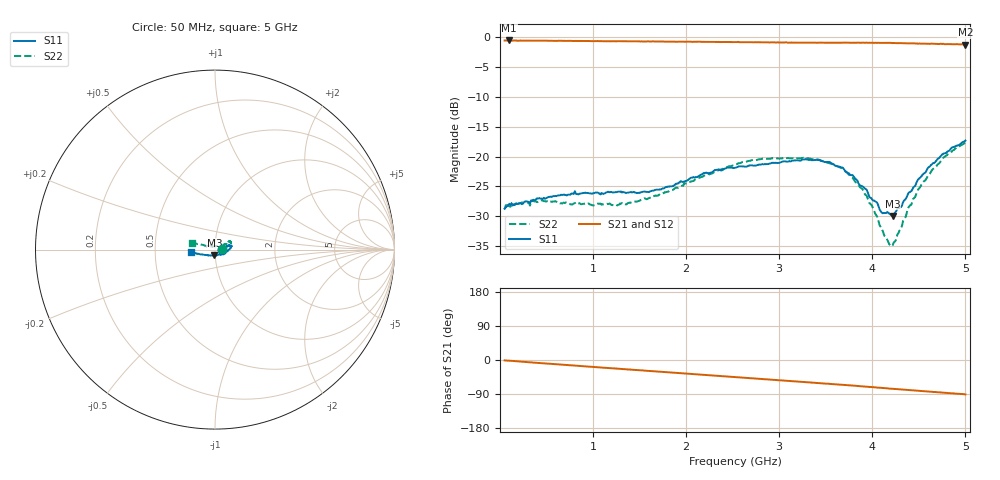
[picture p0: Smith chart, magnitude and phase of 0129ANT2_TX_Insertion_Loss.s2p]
! MASWSS0129 de-embedded Sparameters using port extention method. ANT2 to TX Insertion Loss using 3 volt control
! Board loss is removed and phase length of connector and line length of board are dialed out
! 100pF blocking capacitor
! Sample board 1000013136
#	Hz	S	DB	R	50
!	Freq	S11	S21	S12	S22
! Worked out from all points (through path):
!   401 points, 50 MHz to 5 GHz, reference 50 ohm
!   highest |S21| = -0.52 dB at 99.5 MHz (marker M1); lowest = -1.2 dB at 5 GHz (marker M2)
!   group delay of S21, straight-line fit = 49.8 ps
!   lowest |S11| = -30.0 dB at 4.22 GHz (marker M3), VSWR 1.07, Z = 49.5 - j3.13 ohm
!   |S11| at or under -10 dB: start of sweep to end of sweep
!   |S22| runs from -35.0 to -17.6 dB; largest |S21 - S12| = 0.011
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5e7  -28.76 -0.5  -0.53 -1.0  -0.49 -1.3  -28.81 2.1
9.95e7  -27.92 -0.9  -0.52 -1.8  -0.51 -1.9  -28.36 3.2
4.58e8  -27.14 7.4  -0.55 -8.5  -0.55 -8.7  -27.36 9.9
8.79e8  -26.17 -1.4  -0.61 -16.1  -0.61 -16.1  -27.99 8.5
1.25e9  -25.98 0.2  -0.67 -22.6  -0.66 -22.7  -28.28 11.1
1.7e9  -25.57 10.3  -0.70 -30.5  -0.70 -30.6  -26.54 24.3
2.19e9  -22.77 15.6  -0.75 -39.2  -0.76 -39.3  -23.23 28.2
2.53e9  -21.88 16.0  -0.79 -45.1  -0.80 -45.2  -21.42 30.3
2.82e9  -21.27 14.6  -0.82 -50.3  -0.84 -50.4  -20.37 29.1
3.35e9  -20.62 11.7  -0.89 -59.7  -0.90 -59.8  -20.43 22.8
3.63e9  -21.67 2.3  -0.90 -64.5  -0.90 -64.6  -21.66 22.7
3.79e9  -23.14 -8.5  -0.90 -67.4  -0.91 -67.7  -23.58 27.4
3.94e9  -25.58 -23.4  -0.88 -70.4  -0.92 -70.5  -26.61 34.4
4.05e9  -27.72 -44.9  -0.93 -72.5  -0.93 -72.7  -30.02 47.4
4.11e9  -29.52 -63.0  -0.93 -73.8  -0.94 -73.9  -32.44 60.4
4.18e9  -29.54 -83.6  -0.92 -75.4  -0.93 -75.4  -34.66 87.4
4.22e9  -29.96 -96.7  -0.96 -76.1  -0.95 -76.2  -34.85 105.4
4.31e9  -28.45 -120.8  -0.97 -77.7  -0.99 -77.8  -32.05 139.1
4.39e9  -26.08 -139.8  -1.01 -79.4  -1.01 -79.6  -28.48 151.3
4.55e9  -22.88 -157.0  -1.05 -82.4  -1.05 -82.6  -24.22 159.0
4.76e9  -19.55 -167.2  -1.08 -86.2  -1.14 -86.7  -20.25 161.3
5e9  -17.32 -174.5  -1.20 -90.9  -1.21 -91.0  -17.65 163.9
